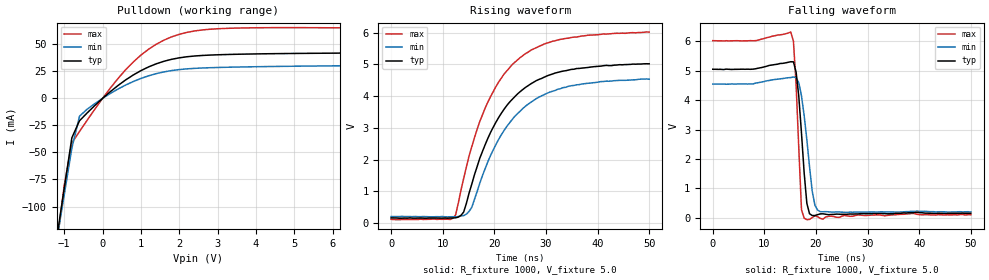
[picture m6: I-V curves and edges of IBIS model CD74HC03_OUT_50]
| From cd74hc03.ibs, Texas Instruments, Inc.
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|   Model CD74HC03 OUTPUT_50
[Model]   CD74HC03_OUT_50
Model_type  Open_drain
Polarity   Non-Inverting
Vref = 5.0
Rref = 1000
Cref = 50p
Vmeas = 2.5
| variable   typ   min   max
C_comp   1.930pf   1.534pf   2.323pf
[Temperature Range]   25   85   -40
[Voltage range]   5.0   4.5   6.0
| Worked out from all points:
|   slope of the pulldown table from 0 to 0.75 V, typ, clamps not added: 36.7 ohm
|   rising waveform, R_fixture 1000, V_fixture 5.0: 20-80 % time 8.9ns typ, 9.11ns min, 8.74ns max; typ from 0.169 V to 5.02 V
|   falling waveform, R_fixture 1000, V_fixture 5.0: 20-80 % time 1.22ns typ, 1.62ns min, 900ps max; typ from 5.05 V to 0.146 V
[Pulldown]
|   Voltage   I(typ)   I(min)   I(max)
-5V       -1.025A    -957.9mA   -1.207A
-1.2V     -130.5mA   -132.8mA   -137mA
-1V       -83.48mA   -89.39mA   -80.63mA
-800mV    -36.41mA   -45.96mA   -41.21mA
-600mV    -20.63mA   -16.42mA   -30.52mA
0V        17.06uA    21.92uA    -17.73uA
600mV     17.03mA    12.3mA     26.4mA
1.2V      29.11mA    20.87mA    45.47mA
1.8V      36.14mA    25.73mA    56.89mA
2.4V      39.2mA     27.77mA    62.36mA
3.4V      40.72mA    28.91mA    64.93mA
10V       43.25mA    31.73mA    64.85mA
[ramp]
| variable   typ   min   max
dV/dt_r   2.981E+00/8.541E-09  2.646E+00/8.760E-09  3.618E+00/8.375E-09
dV/dt_f   3.012E+00/1.125E-09  2.682E+00/1.537E-09  3.363E+00/7.780E-10
[Rising Waveform]
R_fixture = 1000
V_fixture = 5.0
V_fixture_min = 4.5
V_fixture_max = 6.0
C_fixture = 0
L_fixture = 0
|   Time   V(typ)   V(min)   V(max)
0s        169.4mV    211.3mV    123.8mV
11.46ns   165.3mV    204.9mV    118.6mV
12.5ns    171.8mV    201.1mV    262.8mV
14.06ns   352.9mV    242.2mV    1.411V
15.63ns   1.23V      500mV      2.408V
18.23ns   2.475V     1.722V     3.629V
21.88ns   3.586V     2.919V     4.694V
26.04ns   4.275V     3.685V     5.337V
34.38ns   4.82V      4.312V     5.824V
50ns      5.017V     4.532V     6.016V
[Falling Waveform]
R_fixture = 1000
V_fixture = 5.0
V_fixture_min = 4.5
V_fixture_max = 6.0
C_fixture = 0
L_fixture = 0
|   Time   V(typ)   V(min)   V(max)
0s        5.051V     4.546V     6.024V
15.1ns    5.306V     4.768V     6.319V
15.63ns   5.302V     4.787V     6.003V
16.15ns   4.951V     4.766V     4.516V
17.19ns   2.871V     4.144V     270.8mV
17.71ns   1.517V     3.469V     -15.08mV
18.23ns   485.4mV    2.649V     -68.21mV
19.27ns   73.09mV    898.5mV    4.273mV
20.83ns   128.9mV    204mV      -25.18mV
50ns      145.6mV    193.5mV    99.18mV
